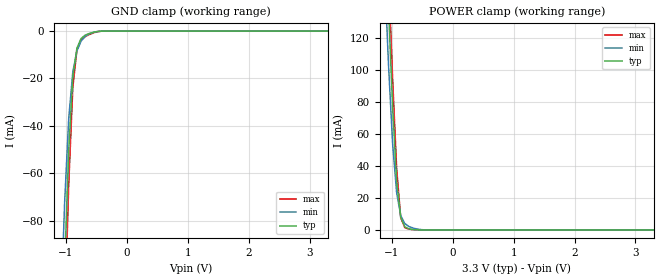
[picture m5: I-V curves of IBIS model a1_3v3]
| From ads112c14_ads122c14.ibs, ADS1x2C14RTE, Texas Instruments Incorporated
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|   Model a1_3v3
[Model] a1_3v3
Model_type Input
Polarity   Non-Inverting
Enable   Active-High
Vinl =  0.990V
Vinh =  2.310V
C_comp   1.600pF   0.800pF   3.200pF
[Model Spec]
Vinh   2.310V   2.100V   2.520V
Vinl   0.990V   0.900V   1.080V
[Temperature Range]   27.000   0.125k   -40.000
[Voltage Range]   3.300V   3.000V   3.600V
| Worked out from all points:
|   GND clamp passes 1 mA (typ) near -0.62 V on its own axis
|   POWER clamp passes 1 mA (typ) near -0.73 V on its own axis
[GND_clamp]
|Voltage   I(typ)   I(min)   I(max)
-3.3V     -2.59A     -2.502A    -2.652A
-1.089V   -157.6mA   -120.4mA   -186.1mA
-1.022V   -98.84mA   -72.04mA   -121.8mA
-955mV    -50.01mA   -36.72mA   -64.56mA
-888mV    -19.26mA   -17.14mA   -23.69mA
-821mV    -7.27mA    -8.43mA    -7.991mA
-754mV    -3.173mA   -4.286mA   -3.815mA
-687mV    -1.72mA    -2.263mA   -2.418mA
-553mV    -529.3uA   -525.6uA   -783uA
-352mV    -4.762uA   -9.213uA   -3.113uA
3.3V      0A         0A         0A
[POWER_clamp]
|Voltage   I(typ)   I(min)   I(max)
-3.3V     2.665A     2.603A     2.705A
-1.122V   207mA      164.3mA    233.9mA
-1.055V   139.2mA    103.8mA    162.8mA
-988mV    77.62mA    54.62mA    95.67mA
-921mV    30.68mA    23.29mA    38.7mA
-854mV    7.996mA    9.08mA     7.692mA
-787mV    2.006mA    4.011mA    1.422mA
-720mV    730.5uA    2.191mA    566uA
-653mV    272.9uA    1.229mA    196.5uA
-452mV    2.05uA     53.78uA    272.3nA
3.3V      0A         0A         0A
